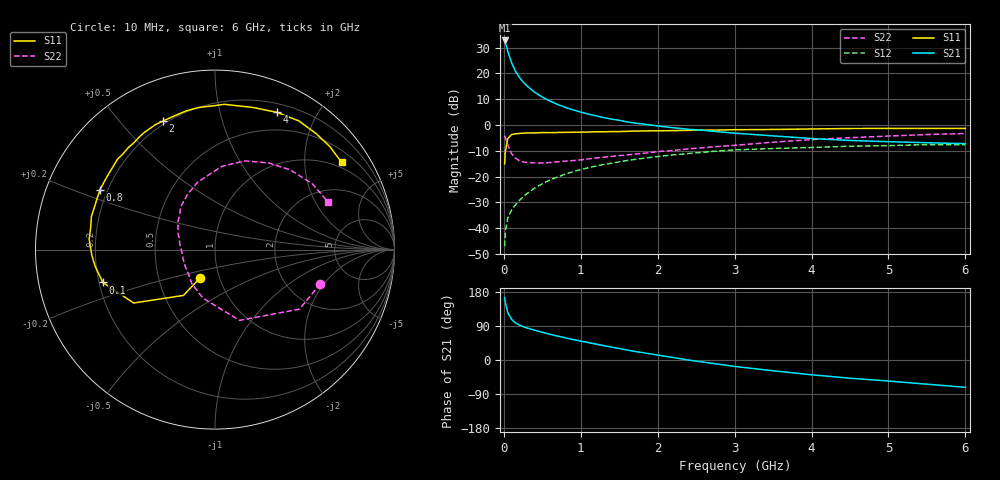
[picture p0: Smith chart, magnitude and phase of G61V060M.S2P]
! SIEMENS Small Signal Semiconductors
! BFG193
! Si NPN RF Bipolar Junction Transistor in SOT223
! VCE = 1 V  IC = 60 mA
! Common Emitter S-Parameters:  August  1996
# GHz  S  MA  R  50
!  f  S11  S21  S12  S22
! GHz  MAG  ANG  MAG  ANG  MAG  ANG  MAG  ANG
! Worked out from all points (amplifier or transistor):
!   36 points, 10 MHz to 6 GHz, reference 50 ohm
!   highest |S21| = 32.8 dB at 10 MHz (marker M1)
!   |S21| within 3 dB of that: start of sweep to 40.2 MHz
!   unconditionally stable (mu >= 1): start of sweep to 17.4 MHz; 160.1 MHz to end of sweep
!   at 250 MHz: K = 1.11, MAG = 20.3 dB, |S12| = -27.9 dB
!   at 1.4 GHz: K = 1.17, MAG = 6.0 dB, |S12| = -14.8 dB
!   at 6 GHz: K = 1.06, MAG = -1.2 dB, |S12| = -7.6 dB
!   S11 on the Smith chart (normalised r, x): 10 MHz: 0.81, -0.26; 100 MHz: 0.22, -0.14; 800 MHz: 0.17, +0.24; 2 GHz: 0.19, +0.66; 4 GHz: 0.29, +1.51; 6 GHz: 0.83, +3.02
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0.01  0.1771 -117.8  43.45 164.9  0.0045 72.9  0.6176 -18.0
0.02  0.3096 -124.5  39.6 152.0  0.0086 67.3  0.5757 -35.2
0.05  0.5419 -146.7  27.21 125.6  0.0157 56.4  0.4174 -70.9
0.1  0.6512 -163.7  16.1 107.5  0.0224 55.9  0.2787 -103.8
0.15  0.6743 -172.1  11.09 98.0  0.0283 58.1  0.2305 -123.8
0.2  0.6868 -177.3  8.49 92.4  0.0344 61.8  0.2037 -135.5
0.25  0.6942 178.9  6.821 88.1  0.0404 63.0  0.1928 -146.6
0.3  0.7035 175.2  5.721 84.6  0.047 63.9  0.1887 -153.2
0.4  0.7033 170.1  4.324 78.8  0.06 65.0  0.1845 -165.1
0.5  0.7131 164.9  3.472 73.0  0.0726 64.1  0.1836 -173.3
0.6  0.712 160.8  2.91 68.0  0.0863 62.8  0.1873 -179.2
0.8  0.7223 152.4  2.194 58.5  0.1118 59.2  0.1997 170.0
1.1  0.7318 141.1  1.627 45.9  0.1489 53.2  0.2208 158.1
1.6  0.7552 124.3  1.151 26.5  0.2052 40.7  0.2637 140.7
2  0.7724 112.2  0.96 13.0  0.2447 30.7  0.3056 128.6
2.2  0.7789 106.8  0.886 6.6  0.2638 25.6  0.3215 122.5
2.8  0.8005 91.1  0.738 -11.3  0.3154 10.6  0.386 104.9
3.5  0.8201 74.9  0.616 -28.4  0.3509 -7.7  0.4649 85.4
4  0.8388 65.7  0.548 -39.0  0.3667 -17.3  0.5219 71.3
4.5  0.8558 56.9  0.502 -48.1  0.3886 -27.2  0.5684 58.1
5.5  0.8597 41.9  0.454 -63.8  0.4176 -49.5  0.6541 34.2
6  0.8569 34.5  0.435 -72.1  0.4146 -62.1  0.684 22.8
